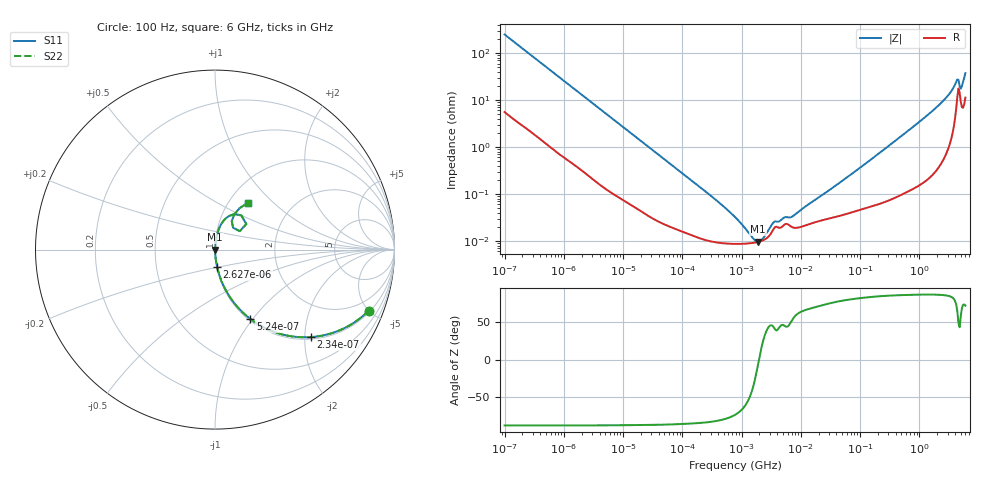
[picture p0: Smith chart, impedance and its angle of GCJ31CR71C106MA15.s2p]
!Murata Part Number: GCJ31CR71C106MA15
!These Parameters are Measured in Series Mode Connection
!Data Generated on Mar 13, 2026
!  o--ll--o
!Port1  Port2
!  o------o
!Operation Temp=25[degC], DC Bias Voltage=0[V]
!Freq. Start=100[Hz] Stop=6[GHz] 401[Steps]
# Hz S RI R 50
!Freq.(Hz) S11(Real) S11(Imag) S21(Real) S21(Imag) S12(Real) S12(Imag) S22(Real) S22(Imag)
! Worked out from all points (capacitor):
!   401 points, 100 Hz to 6 GHz, reference 50 ohm
!   read as one part in series: C = 6.36 uF near 109 Hz
!   lowest |Z| = 9.61 mohm at 1.897 MHz (marker M1)
!   series resonance near 1.97 MHz, so ESL is about 1 nH
!   S11 on the Smith chart (normalised r, x): 100 Hz: 1.11, -4.98; 234 Hz: 1.05, -2.15; 524 Hz: 1.02, -0.97; 2.627 kHz: 1.00, -0.20; 6 GHz: 1.22, +0.72
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100  0.8557 -0.3405  0.1443 0.3405  0.1443 0.3405  0.8557 -0.3405
150  0.7322 -0.4318  0.2678 0.4318  0.2678 0.4318  0.7322 -0.4318
234  0.5357 -0.4874  0.4643 0.4874  0.4643 0.4874  0.5357 -0.4874
524  0.1968 -0.3863  0.8032 0.3863  0.8032 0.3863  0.1968 -0.3863
938  0.0748 -0.2518  0.9252 0.2518  0.9252 0.2518  0.0748 -0.2518
2008  0.0195 -0.1265  0.9805 0.1265  0.9805 0.1265  0.0195 -0.1265
2627  0.0121 -0.0979  0.9879 0.0979  0.9879 0.0979  0.0121 -0.0979
40335  0.0003 -0.00674  0.9997 0.00674  0.9997 0.00674  0.0003 -0.00674
302498  9.89e-05 -0.000913  0.9999 0.000913  0.9999 0.000913  9.89e-05 -0.000913
774597  8.67e-05 -0.000311  0.9999 0.000311  0.9999 0.000311  8.67e-05 -0.000311
1585629  9.12e-05 -6.45e-05  0.9999 6.45e-05  0.9999 6.45e-05  9.12e-05 -6.45e-05
1896632  9.54e-05 -1.13e-05  0.9999 1.13e-05  0.9999 1.13e-05  9.54e-05 -1.13e-05
2268635  0.000103 4.3e-05  0.9999 -4.3e-05  0.9999 -4.3e-05  0.000103 4.3e-05
3549919  0.000188 0.000173  0.9998 -0.000173  0.9998 -0.000173  0.000188 0.000173
7266822  0.000195 0.000271  0.9998 -0.000271  0.9998 -0.000271  0.000195 0.000271
1.555665e7  0.00024 0.000639  0.9998 -0.000639  0.9998 -0.000639  0.00024 0.000639
3.124326e8  0.000853 0.0108  0.9991 -0.0108  0.9991 -0.0108  0.000853 0.0108
1.369159e9  0.00425 0.0472  0.9957 -0.0472  0.9957 -0.0472  0.00425 0.0472
2.802721e9  0.0185 0.1072  0.9815 -0.1072  0.9815 -0.1072  0.0185 0.1072
4.193612e9  0.1046 0.1969  0.8954 -0.1969  0.8954 -0.1969  0.1046 0.1969
5.245841e9  0.0936 0.1589  0.9064 -0.1589  0.9064 -0.1589  0.0936 0.1589
6e9  0.1856 0.2623  0.8144 -0.2623  0.8144 -0.2623  0.1856 0.2623
